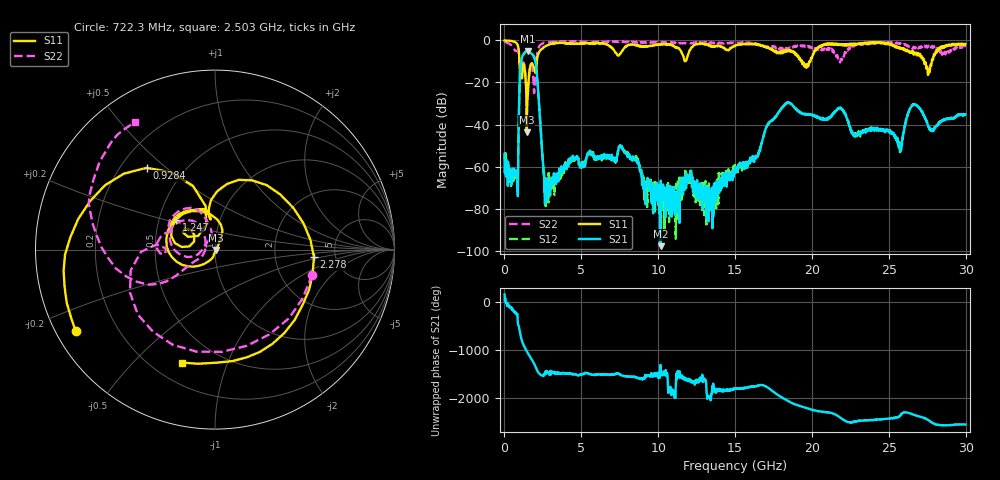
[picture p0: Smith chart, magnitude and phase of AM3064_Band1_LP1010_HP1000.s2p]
# Hz S DB R 50.0
!freq dBS11 angS11 dBS21 angS21 dBS12 angS12 dBS22 angS22
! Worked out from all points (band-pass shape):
!   1600 points, 10 MHz to 29.98 GHz, reference 50 ohm
!   highest |S21| = -5.06 dB at 1.51 GHz (marker M1); lowest = -97.7 dB at 10.15 GHz (marker M2)
!   |S21| within 3 dB of the highest: 1.138 GHz to 1.934 GHz (795.6 MHz wide, 51.8 % of centre)
!   lowest |S11| = -43.7 dB at 1.453 GHz (marker M3), VSWR 1.01, Z = 50.6 - j0.181 ohm
!   |S11| at or under -10 dB: 973.8 MHz to 2.106 GHz (1.132 GHz wide, 73.5 % of centre); 19.36 GHz to 19.84 GHz (477.5 MHz wide, 2.44 % of centre); 27.3 GHz to 27.8 GHz (495.6 MHz wide, 1.8 % of centre)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
!   |S22| runs from -25.1 to -0.4 dB; largest |S21 - S12| = 0.0073
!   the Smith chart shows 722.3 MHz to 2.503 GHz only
!   S11 on the Smith chart (normalised r, x): 722.3 MHz: 0.06, -0.27; 928.4 MHz: 0.31, +0.43; 1.247 GHz: 0.61, +0.22; 2.278 GHz: 3.42, -0.40; 2.503 GHz: 0.32, -0.70
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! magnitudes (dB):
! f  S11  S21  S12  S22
! 10 MHz  0.0  -53.8  -54.2  -0.4
! 722.3 MHz  -0.9  -61.8  -61.7  -5.0
! 928.4 MHz  -4.5  -39.3  -39.4  -6.3
! 1.247 GHz  -11.3  -6.5  -6.4  -10.6
! 1.453 GHz  -43.7  -5.1  -5.1  -23.9
! 1.51 GHz  -26.9  -5.1  -5.0  -23.7
! 1.978 GHz  -14.6  -9.0  -9.0  -19.9
! 2.278 GHz  -5.2  -33.3  -33.3  -2.5
! 2.503 GHz  -3.7  -57.4  -58.6  -1.5
! 2.784 GHz  -2.3  -65.5  -69.5  -1.0
! 5.015 GHz  -1.4  -58.6  -59.7  -0.6
! 7.582 GHz  -5.9  -50.2  -50.4  -0.5
! 10 GHz  -2.0  -74.8  -72.9  -0.9
! 10.15 GHz  -1.9  -97.7  -78.1  -1.0
! 15 GHz  -2.5  -63.0  -63.5  -1.4
! 18.32 GHz  -5.4  -30.1  -30.0  -3.6
! 19.99 GHz  -8.5  -35.3  -35.5  -3.2
! 25 GHz  -1.4  -43.3  -43.2  -1.1
! 25.75 GHz  -3.5  -52.2  -52.2  -1.6
! 26.64 GHz  -6.4  -30.4  -30.6  -3.4
! 27.56 GHz  -16.3  -41.0  -40.6  -2.7
! 29.98 GHz  -1.8  -35.2  -34.9  -3.2
